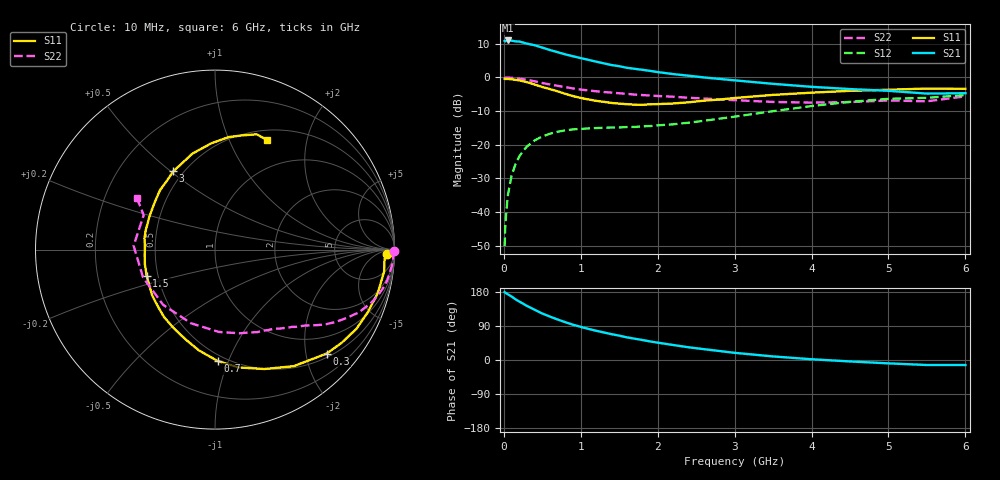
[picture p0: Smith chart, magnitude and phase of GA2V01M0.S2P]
! Infineon Technologies  Discrete & RF Semiconductors
! BF775
! Si NPN RF Bipolar Junction Transistor in SOT23
! VCE = 2 V  IC = 1 mA
! Common Emitter S-Parameters:  May  1996
# GHz  S  MA  R  50
!  f  S11  S21  S12  S22
! GHz  MAG  ANG  MAG  ANG  MAG  ANG  MAG  ANG
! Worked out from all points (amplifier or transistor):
!   36 points, 10 MHz to 6 GHz, reference 50 ohm
!   highest |S21| = 11.0 dB at 50 MHz (marker M1)
!   |S21| within 3 dB of that: start of sweep to 623.3 MHz
!   unconditionally stable (mu >= 1): 1.397 GHz to end of sweep
!   at 250 MHz: K = 0.21, MSG = 16.1 dB, |S12| = -21.9 dB
!   at 1.4 GHz: K = 1.00, MAG = 9.0 dB, |S12| = -14.9 dB
!   at 6 GHz: K = 1.05, MAG = -1.1 dB, |S12| = -5.3 dB
!   S11 on the Smith chart (normalised r, x): 10 MHz: 33, -19; 300 MHz: 0.58, -2.43; 700 MHz: 0.45, -0.91; 1.5 GHz: 0.43, -0.15; 3 GHz: 0.44, +0.51; 6 GHz: 0.62, +1.39
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0.01  0.9559 -1.5  3.493 179.1  0.0031 90.5  0.9988 -0.6
0.02  0.9462 -3.1  3.437 177.4  0.0067 87.6  0.9912 -1.3
0.05  0.9502 -7.4  3.54 173.8  0.0171 85.6  0.9954 -3.4
0.1  0.9386 -15.0  3.512 167.6  0.0344 81.6  0.9846 -6.8
0.15  0.9199 -22.3  3.438 160.4  0.0507 76.0  0.9746 -10.1
0.2  0.9034 -29.2  3.411 154.5  0.0665 71.7  0.9593 -13.2
0.3  0.8505 -42.9  3.174 142.7  0.0939 64.0  0.9196 -18.8
0.4  0.7836 -56.0  3.006 132.7  0.1158 56.8  0.8741 -23.6
0.5  0.7197 -67.6  2.771 122.6  0.1324 50.9  0.8243 -27.6
0.7  0.6204 -88.7  2.367 106.8  0.1558 41.8  0.7492 -33.6
0.9  0.5267 -108.1  2.06 93.1  0.1688 36.0  0.6855 -38.0
1.1  0.4704 -127.3  1.822 82.1  0.1746 32.3  0.6389 -41.9
1.3  0.4336 -143.7  1.616 72.7  0.1789 30.3  0.6061 -45.3
1.5  0.4075 -159.1  1.467 64.3  0.1804 29.7  0.5808 -48.8
1.9  0.3981 170.8  1.251 49.0  0.1889 32.1  0.5376 -56.5
2.2  0.4095 153.0  1.121 39.6  0.2007 34.2  0.5161 -63.0
3  0.4941 118.1  0.904 18.9  0.261 38.3  0.459 -87.4
3.5  0.5495 103.2  0.802 9.4  0.3147 36.5  0.4316 -108.0
4.5  0.6315 83.1  0.67 -3.8  0.4335 25.4  0.4298 -158.9
5  0.655 76.4  0.632 -8.9  0.4801 17.7  0.4539 177.3
5.5  0.683 70.1  0.574 -13.2  0.4972 9.1  0.4414 154.2
6  0.676 64.6  0.582 -13.3  0.5454 4.6  0.5223 146.5
